(* Logix 5000 AddOnInstructionDefinition export Banner_TLF100_PD_v2; software revision 32.00 *)

TYPE Banner_TLF100_Adv_PD_Seg_v2 :   // Advanced process data set for a TLF100 Segment.
STRUCT
   Animation_Type : SINT;   // 0 = Off, 1 = Steady, 2 = Flash, 3 = Two Color Flash, 4 = 2Color Shift, 5 = Ends Steady, 6 = Ends Flash, 7 = Scroll, 8 = Center Scroll, 9 = Bounce, 10 = Center Bounce, 11 = Intensity Sweep, 12 = Two Color Sweep, 13 = Spectrum, 14 = Level Steady, 15 = Level Flash
   Color_1 : SINT;   // 0 = Green, 1 = Red, 2 = Orange, 3 = Amber, 4 = Yellow, 5 = Lime Green, 6 = Spring Green, 7 = Cyan, 8 = Sky Blue, 9 = Blue, 10 = Violet, 11 = Magenta, 12 = Rose, 13 = White, 14 = Custom, 15 = Custom 2
   Color_1_Intensity : SINT;   // 0 = High, 1 = Low, 2 = Medium, 3 = Off, 4 = Custom
   Color_2 : SINT;   // 0 = Green, 1 = Red, 2 = Orange, 3 = Amber, 4 = Yellow, 5 = Lime Green, 6 = Spring Green, 7 = Cyan, 8 = Sky Blue, 9 = Blue, 10 = Violet, 11 = Magenta, 12 = Rose, 13 = White, 14 = Custom, 15 = Custom 2
   Color_2_Intensity : SINT;   // 0 = High, 1 = Low, 2 = Medium, 3 = Off, 4 = Custom
   Speed : SINT;   // 0 = Medium, 1 = Fast, 2 = Slow, 3 = Custom
   Pulse_Pattern : SINT;   // 0 = Normal, 1 = Strobe, 2 = Three Pulse, 3 = SOS, 4 = Random
   Scroll_Bounce : SINT;   // 0 = Solid, 1 = Tail, 2 = Ripple
   Direction : SINT;   // 0 = up, 1 = down
   Percent_Width_of_C1 : SINT;   // 1 to 100 %
END_STRUCT
END_TYPE

TYPE Banner_TLF100_Adv_PDIO_v2 :   // Advanced process data set for a TLF100 IO-Link unit.
STRUCT
   Segment_1 : Banner_TLF100_Adv_PD_Seg_v2;   // Advanced process data set for a TL70 Segment.
   Segment_2 : Banner_TLF100_Adv_PD_Seg_v2;   // Advanced process data set for a TL70 Segment.
   Segment_3 : Banner_TLF100_Adv_PD_Seg_v2;   // Advanced process data set for a TL70 Segment.
   Segment_4 : Banner_TLF100_Adv_PD_Seg_v2;   // Advanced process data set for a TL70 Segment.
   Audible : SINT;   // 0 = Pulse, 1 = Wobble, 2 = Strobe, 4 = Whoop, 5 = Stacatto, 6 = Siren, 8 = Continuous 1, 9 = Continuous 2, 16 = Jingle, 17 = Melody 1, 18 = Melody 2, 19 = Melody 3, 20 = Custom
   Audible_Volume : SINT;   // 0 = Off, 1 = Low, 2 = Medium, 3 = High
END_STRUCT
END_TYPE

TYPE Banner_TLF100_Level_PD_v2 :   // LeveL process data set for a TLF100 Pro IO-Link unit.
STRUCT
   Level_Mode_Value : DINT;   // Value describing the level of the device. Range determined in Level Mode Parameter.
END_STRUCT
END_TYPE

TYPE Banner_TLF100_PDIO_v2 :   // Process data for a Banner TLF100 unit. This includes four process data types.
STRUCT
   Segment_PD : Banner_TLF100_Segment_PD_v2;
   Run_PD : Banner_TLF100_Run_PD_v2;
   Level_PD : Banner_TLF100_Level_PD_v2;
   Advanced_PD : Banner_TLF100_Adv_PDIO_v2;
   Transfer_Data : SINT[31];   // Data array to send teh correct state of the process data output to the IO-Link master.
END_STRUCT
END_TYPE

TYPE Banner_TLF100_Run_PD_v2 :   // Run mode process data set for a TLF100 Pro IO-Link unit.
STRUCT
   Animation : SINT;   // 0 = Off, 1 = Steady, 2 = Flash, 3 = Two Color, 4 = Half/Half, 5 = Half/Half Rotate, 6 = Chase, 7 = Intesnity Sweep, 8 = Scroll, 9 = Bounce, 10 = Demo
   Color_1 : SINT;   // 0 = Green, 1 = Red, 2 = Orange, 3 = Amber, 4 = Yellow, 5 = Lime Green, 6 = Spring Green, 7 = Cyan, 8 = Sky Blue, 9 = Blue, 10 = Violet, 11 = Magenta, 12 = Rose, 13 = White, 14 = Custom, 15 = Custom 2
   Color_1_Intensity : SINT;   // 0 = High, 1 = Low, 2 = Medium, 3 = Off, 4 = Custom
   Color_2 : SINT;   // 0 = Green, 1 = Red, 2 = Orange, 3 = Amber, 4 = Yellow, 5 = Lime Green, 6 = Spring Green, 7 = Cyan, 8 = Sky Blue, 9 = Blue, 10 = Violet, 11 = Magenta, 12 = Rose, 13 = White, 14 = Custom, 15 = Custom 2
   Color_2_Intensity : SINT;   // 0 = High, 1 = Low, 2 = Medium, 3 = Off, 4 = Custom
   Speed : SINT;   // 0 = Medium, 1 = Fast, 2 = Slow, 3 = Custom
   Pulse_Pattern : SINT;   // 0 = Normal, 1 = Strobe, 2 = Three Pulse, 3 = SOS, 4 = Random
   Direction : SINT;   // 0 = Up, 1 = Down
   Width_of_Color_1 : SINT;   // 1 to 100 percent
   Audible : SINT;   // 0 = Pulse, 1 = Wobble, 2 = Strobe, 4 = Whoop, 5 = Stacatto, 6 = Siren, 8 = Continuous 1, 9 = Continuous 2, 16 = Jingle, 17 = Melody 1, 18 = Melody 2, 19 = Melody 3, 20 = Custom
   Audible_Volume : SINT;   // 0 = Off, 1 = Low, 2 = Medium, 3 = High
END_STRUCT
END_TYPE

TYPE Banner_TLF100_Segment_PD_v2 :   // Basic process data set for a TLF100 IO-Link unit.
STRUCT
   Segment_1 : SINT;   // 0 = Off, 1 = On, 2 = Flash, 3 = Animation Type
   Segment_2 : SINT;   // 0 = Off, 1 = On, 2 = Flash, 3 = Animation Type
   Segment_3 : SINT;   // 0 = Off, 1 = On, 2 = Flash, 3 = Animation Type
   Segment_4 : SINT;   // 0 = Off, 1 = On, 2 = Flash, 3 = Animation Type
   Audible : SINT;   // 0 = Off, 1 = On
END_STRUCT
END_TYPE

ADD_ON_INSTRUCTION Banner_TLF100_Adv_PD_v2   (* revision 2.0, vendor Banner Engineering *)
// AOI converts the Advanced process and places it into the correct bytes for transfer to the IO-Link master.
VAR_IN_OUT
   Segment : Banner_TLF100_Adv_PD_Seg_v2; {required}
   Byte_1 : SINT; {required}
   Byte_2 : SINT; {required}
   Byte_3 : SINT; {required}
   Byte_4 : SINT; {required}
   Byte_5 : SINT; {required}
END_VAR

ROUTINE Logic   (* ladder *)
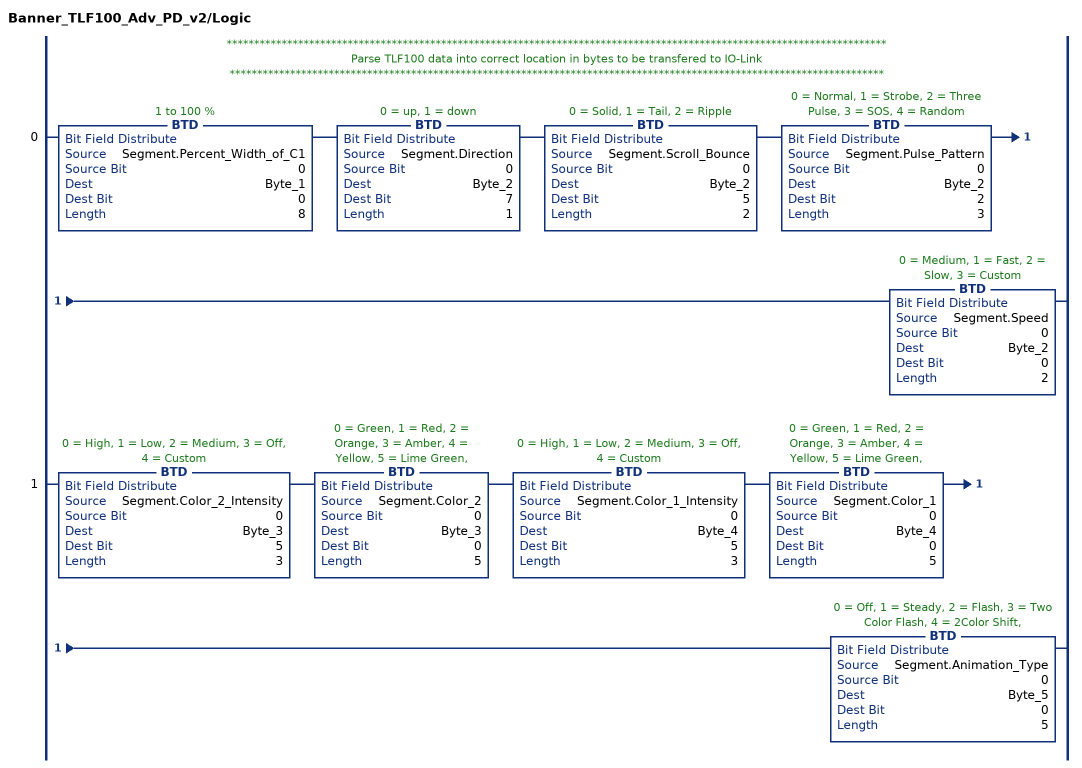
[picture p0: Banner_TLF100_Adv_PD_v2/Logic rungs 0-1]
   // ************************************************************************************************************************
   // Parse TLF100 data into correct location in bytes to be transfered to IO-Link
   // ***********************************************************************************************************************
   0: BTD(Segment.Percent_Width_of_C1,0,Byte_1,0,8)BTD(Segment.Direction,0,Byte_2,7,1)BTD(Segment.Scroll_Bounce,0,Byte_2,5,2)BTD(Segment.Pulse_Pattern,0,Byte_2,2,3)BTD(Segment.Speed,0,Byte_2,0,2);
   1: BTD(Segment.Color_2_Intensity,0,Byte_3,5,3)BTD(Segment.Color_2,0,Byte_3,0,5)BTD(Segment.Color_1_Intensity,0,Byte_4,5,3)BTD(Segment.Color_1,0,Byte_4,0,5)BTD(Segment.Animation_Type,0,Byte_5,0,5);
END_ROUTINE
END_ADD_ON_INSTRUCTION

ADD_ON_INSTRUCTION Banner_TLF100_PD_v2   (* revision 2.1, vendor Banner Engineering *)
// Takes the raw SINT information and converts that data into actual information.
VAR_IN_OUT
   PDIO : Banner_TLF100_PDIO_v2; {required}
END_VAR
VAR_INPUT
   Byte_Swap : BOOL; {required}   // Swap the LSB and the MSB with each other.
   Operation_Mode : INT; {required}   // 0 = Segment, 1 = Run, 2 = Level, 3 = Gauge, 4 = Advanced
END_VAR
VAR
   Temp_Measurement : DINT; {access None}
   Data_Byte : SINT[22]; {access None}
   Temp_Data : SINT[22]; {access None}
   AOI_Status : Banner_TLF100_Adv_PD_v2[10]; {access None}
END_VAR

ROUTINE Logic   (* ladder *)
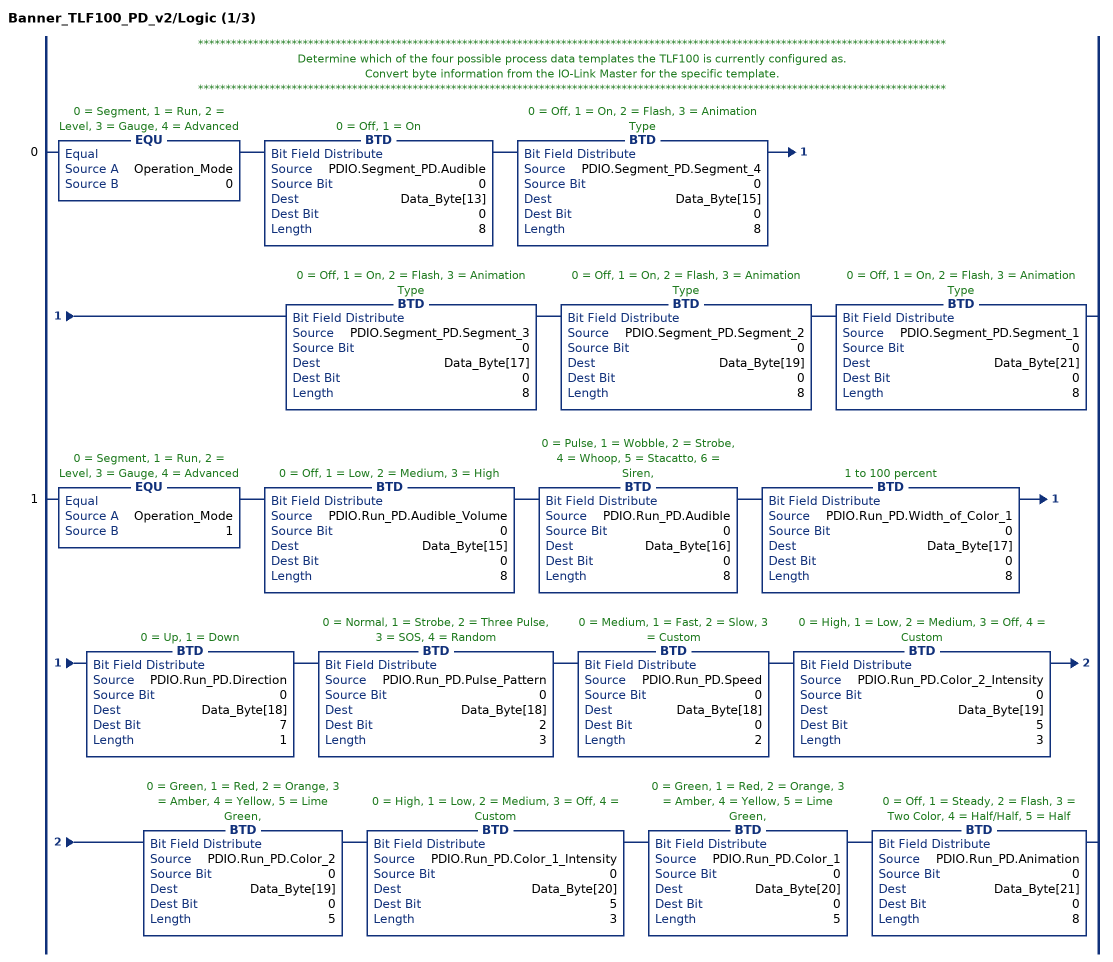
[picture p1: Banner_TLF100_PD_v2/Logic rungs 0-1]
   // ****************************************************************************************************************************************
   // Determine which of the four possible process data templates the TLF100 is currently configured as.
   // Convert byte information from the IO-Link Master for the specific template.
   // ****************************************************************************************************************************************
   0: EQU(Operation_Mode,0)BTD(PDIO.Segment_PD.Audible,0,Data_Byte[13],0,8)BTD(PDIO.Segment_PD.Segment_4,0,Data_Byte[15],0,8)BTD(PDIO.Segment_PD.Segment_3,0,Data_Byte[17],0,8)BTD(PDIO.Segment_PD.Segment_2,0,Data_Byte[19],0,8)BTD(PDIO.Segment_PD.Segment_1,0,Data_Byte[21],0,8);
   1: EQU(Operation_Mode,1)BTD(PDIO.Run_PD.Audible_Volume,0,Data_Byte[15],0,8)BTD(PDIO.Run_PD.Audible,0,Data_Byte[16],0,8)BTD(PDIO.Run_PD.Width_of_Color_1,0,Data_Byte[17],0,8)BTD(PDIO.Run_PD.Direction,0,Data_Byte[18],7,1)BTD(PDIO.Run_PD.Pulse_Pattern,0,Data_Byte[18],2,3)BTD(PDIO.Run_PD.Speed,0,Data_Byte[18],0,2)BTD(PDIO.Run_PD.Color_2_Intensity,0,Data_Byte[19],5,3)BTD(PDIO.Run_PD.Color_2,0,Data_Byte[19],0,5)BTD(PDIO.Run_PD.Color_1_Intensity,0,Data_Byte[20],5,3)BTD(PDIO.Run_PD.Color_1,0,Data_Byte[20],0,5)BTD(PDIO.Run_PD.Animation,0,Data_Byte[21],0,8);
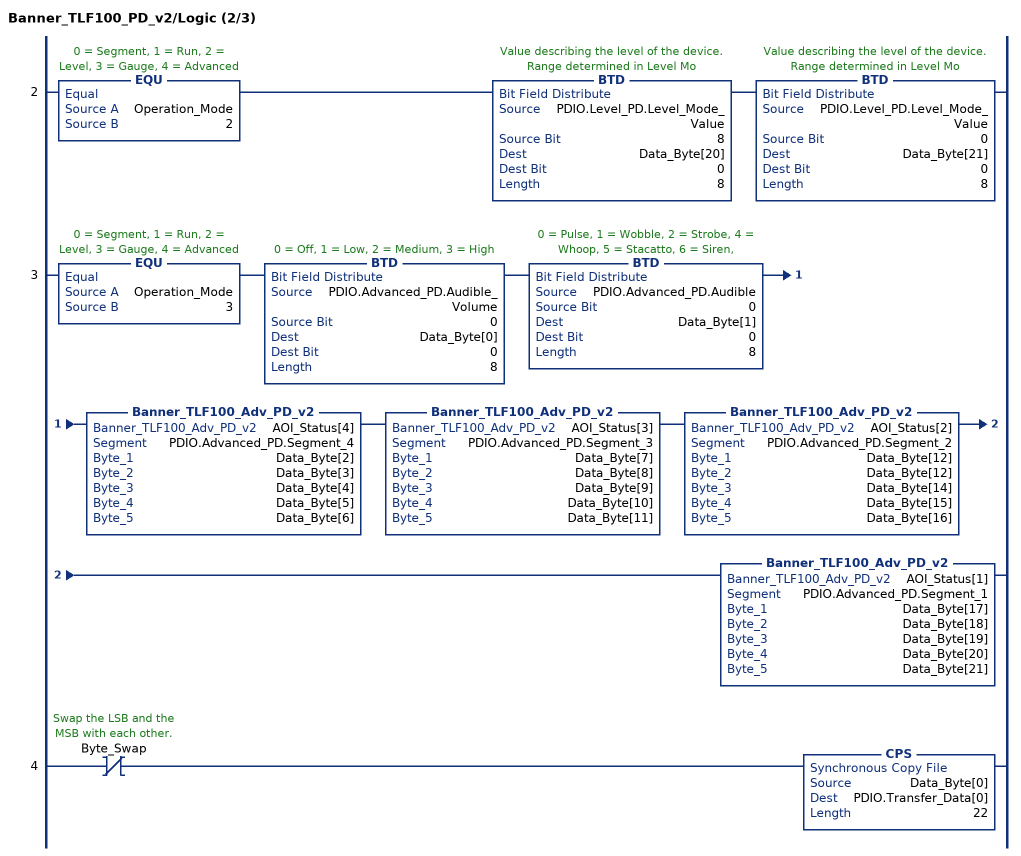
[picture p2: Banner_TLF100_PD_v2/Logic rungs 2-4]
   2: EQU(Operation_Mode,2)BTD(PDIO.Level_PD.Level_Mode_Value,8,Data_Byte[20],0,8)BTD(PDIO.Level_PD.Level_Mode_Value,0,Data_Byte[21],0,8);
   3: EQU(Operation_Mode,3)BTD(PDIO.Advanced_PD.Audible_Volume,0,Data_Byte[0],0,8)BTD(PDIO.Advanced_PD.Audible,0,Data_Byte[1],0,8)Banner_TLF100_Adv_PD_v2(AOI_Status[4],PDIO.Advanced_PD.Segment_4,Data_Byte[2],Data_Byte[3],Data_Byte[4],Data_Byte[5],Data_Byte[6])Banner_TLF100_Adv_PD_v2(AOI_Status[3],PDIO.Advanced_PD.Segment_3,Data_Byte[7],Data_Byte[8],Data_Byte[9],Data_Byte[10],Data_Byte[11])Banner_TLF100_Adv_PD_v2(AOI_Status[2],PDIO.Advanced_PD.Segment_2,Data_Byte[12],Data_Byte[12],Data_Byte[14],Data_Byte[15],Data_Byte[16])Banner_TLF100_Adv_PD_v2(AOI_Status[1],PDIO.Advanced_PD.Segment_1,Data_Byte[17],Data_Byte[18],Data_Byte[19],Data_Byte[20],Data_Byte[21]);
   4: XIO(Byte_Swap)CPS(Data_Byte[0],PDIO.Transfer_Data[0],22);
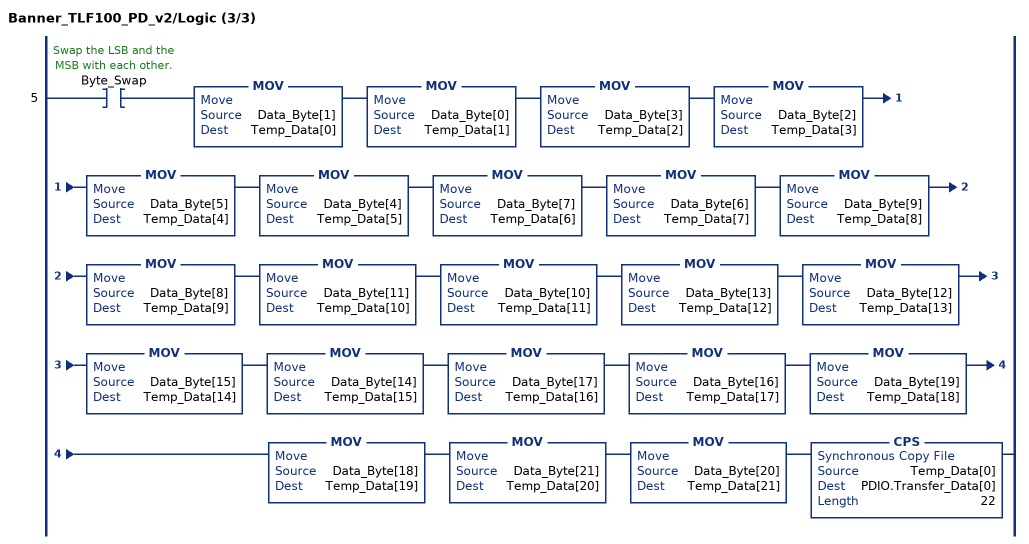
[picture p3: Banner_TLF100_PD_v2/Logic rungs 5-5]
   5: XIC(Byte_Swap)MOV(Data_Byte[1],Temp_Data[0])MOV(Data_Byte[0],Temp_Data[1])MOV(Data_Byte[3],Temp_Data[2])MOV(Data_Byte[2],Temp_Data[3])MOV(Data_Byte[5],Temp_Data[4])MOV(Data_Byte[4],Temp_Data[5])MOV(Data_Byte[7],Temp_Data[6])MOV(Data_Byte[6],Temp_Data[7])MOV(Data_Byte[9],Temp_Data[8])MOV(Data_Byte[8],Temp_Data[9])MOV(Data_Byte[11],Temp_Data[10])MOV(Data_Byte[10],Temp_Data[11])MOV(Data_Byte[13],Temp_Data[12])MOV(Data_Byte[12],Temp_Data[13])MOV(Data_Byte[15],Temp_Data[14])MOV(Data_Byte[14],Temp_Data[15])MOV(Data_Byte[17],Temp_Data[16])MOV(Data_Byte[16],Temp_Data[17])MOV(Data_Byte[19],Temp_Data[18])MOV(Data_Byte[18],Temp_Data[19])MOV(Data_Byte[21],Temp_Data[20])MOV(Data_Byte[20],Temp_Data[21])CPS(Temp_Data[0],PDIO.Transfer_Data[0],22);
END_ROUTINE
END_ADD_ON_INSTRUCTION
